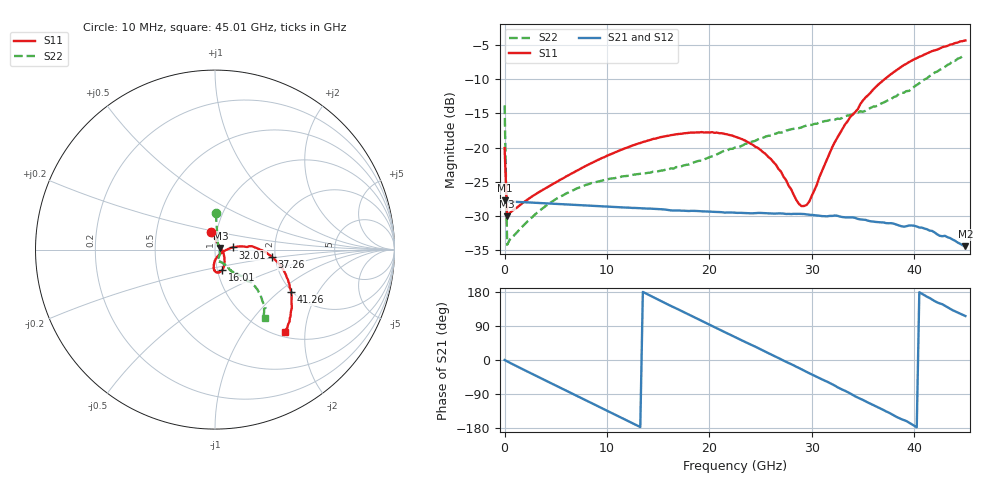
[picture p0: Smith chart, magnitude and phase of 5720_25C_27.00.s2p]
! Device:  ADRF5720
! Description: 0.5dB LSB GaAs MMIC 6-bit Digital Attenuator
! Frequency:  0.000009 -  40 GHz
! Ports:
!	RF1	= Port 1
!	RF2	= Port 2
! Vdd:  3.3 Volt
! Vss:  -3.3 Volt
! Control:  0/3.3 Volt
! State:  27.00 dB attenuation
! Data:  The device was measured using G-S-G Probes on a matrix board.
!  Data was collected using an calibrated 4 port network analyzer.
!  The reference plane for this measurement is at the launchers.
! Note:  Analog Devices supplies this data as a sample of measured data
!  for this product.  Your particular data for this product may vary.
!  Data was taken at 25 degrees C.
!  Analog Devices reserves the right to change this data at anytime.
# GHZ S DB R 45.0
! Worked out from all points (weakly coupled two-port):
!   181 points, 10 MHz to 45.01 GHz, reference 45 ohm
!   highest |S21| = -27.66 dB at 10 MHz (marker M1); lowest = -34.4 dB at 45.01 GHz (marker M2)
!   lowest |S11| = -30.0 dB at 260 MHz (marker M3), VSWR 1.07, Z = 47.8 + j0.882 ohm
!   |S11| at or under -10 dB: start of sweep to 37.16 GHz
!   |S22| runs from -34.2 to -6.5 dB; largest |S21 - S12| = 0.00011
!   S11 on the Smith chart (normalised r, x): 10 MHz: 0.94, +0.18; 16.01 GHz: 1.05, -0.25; 32.01 GHz: 1.22, +0.03; 37.26 GHz: 1.92, -0.18; 41.26 GHz: 1.97, -1.22; 45.01 GHz: 1.09, -1.57
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0.01  -20.07 103.8  -27.66 0.0  -27.66 0.1  -13.86 88.8
0.26  -30.01 17.0  -27.85 -3.7  -27.86 -3.7  -34.17 25.0
3.51  -26.37 -18.1  -28.08 -47.5  -28.08 -47.5  -29.10 -41.1
7.76  -22.81 -43.2  -28.42 -103.8  -28.42 -103.8  -25.55 -69.9
12.01  -19.97 -59.2  -28.75 -160.2  -28.75 -160.2  -24.13 -76.4
15.26  -18.48 -69.1  -28.99 155.9  -28.99 155.9  -23.37 -72.5
16.01  -18.28 -71.4  -29.11 145.8  -29.11 145.8  -23.22 -71.0
20.26  -17.76 -83.6  -29.36 89.8  -29.37 89.8  -21.28 -60.1
22.76  -18.54 -91.1  -29.52 57.2  -29.52 57.3  -19.97 -56.2
24.76  -20.07 -94.1  -29.53 31.6  -29.53 31.6  -18.81 -54.4
26.01  -21.66 -94.2  -29.60 15.0  -29.60 15.0  -18.27 -54.2
27.01  -23.53 -91.4  -29.60 1.8  -29.59 1.9  -17.83 -53.8
29.01  -28.54 -54.5  -29.68 -24.7  -29.68 -24.6  -17.06 -53.9
29.51  -28.36 -37.0  -29.74 -31.7  -29.75 -31.7  -16.79 -52.8
30.26  -26.23 -11.3  -29.85 -41.4  -29.85 -41.4  -16.55 -52.9
32.01  -19.94 7.0  -29.96 -63.9  -29.97 -63.9  -15.97 -51.8
33.26  -16.63 6.9  -30.17 -81.3  -30.16 -81.3  -15.43 -49.4
35.01  -13.14 3.4  -30.50 -105.5  -30.51 -105.4  -14.79 -47.8
37.26  -9.88 -7.4  -31.01 -135.6  -31.01 -135.6  -13.27 -43.8
37.76  -9.29 -10.1  -31.02 -142.2  -31.02 -142.1  -12.95 -43.2
41.26  -6.28 -29.2  -31.91 167.0  -31.91 167.2  -9.91 -43.0
45.01  -4.40 -49.8  -34.37 116.0  -34.38 115.9  -6.53 -53.8
